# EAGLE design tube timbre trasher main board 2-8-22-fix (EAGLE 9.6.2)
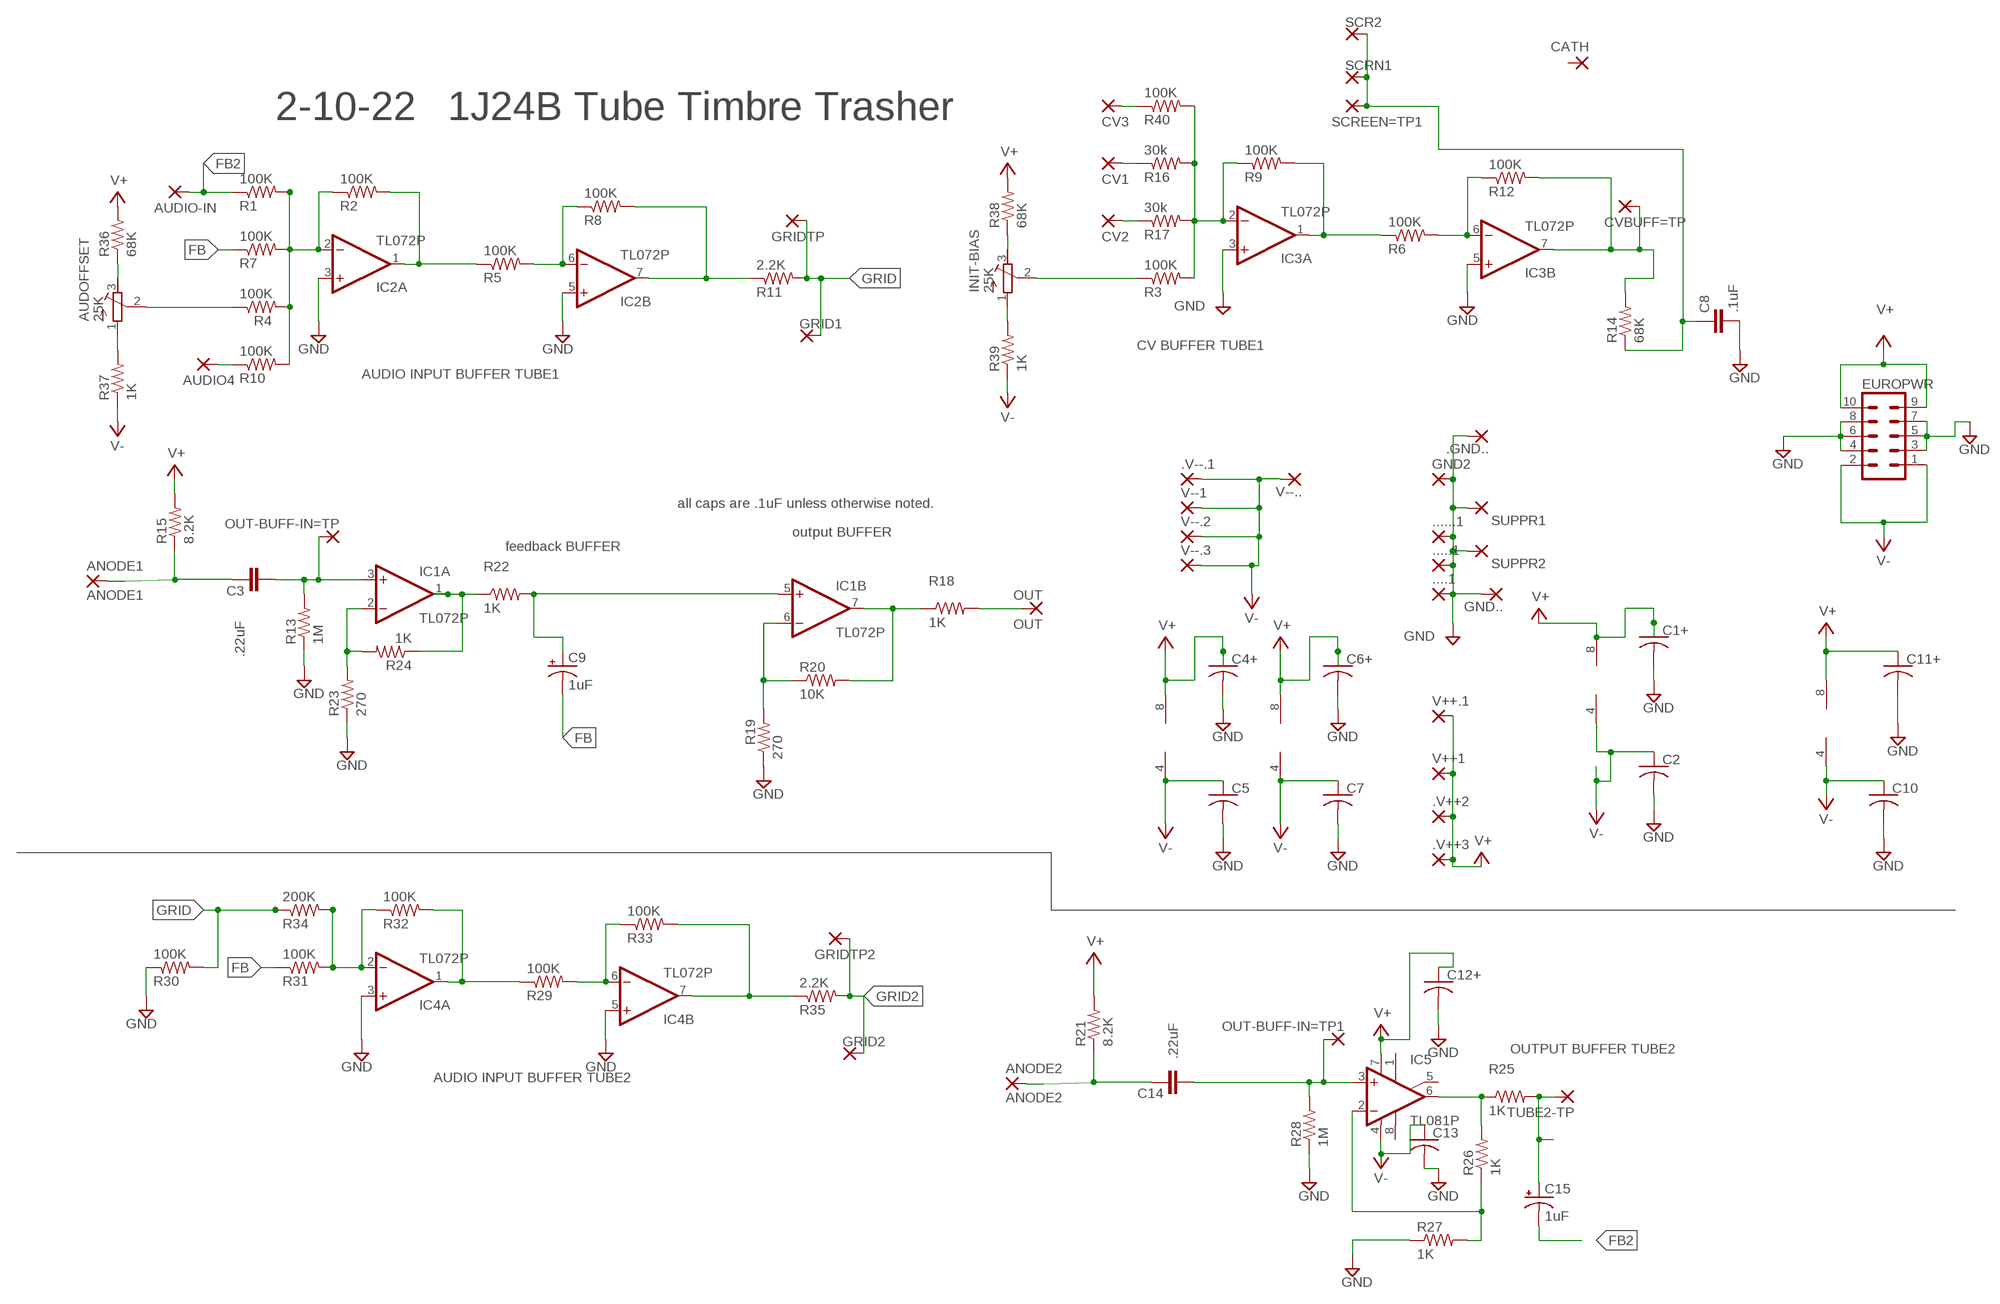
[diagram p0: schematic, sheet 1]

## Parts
....1  3,17/1,3  [3,17/1,3]
.....1  3,17/1,3  [3,17/1,3]
......1  3,17/1,3  [3,17/1,3]
.GND..  1  WIREPAD1,6/0,9  [1,6/0,9]
.V++2  2,54/1,0  [2,54/1,0]
.V++3  2,54/1,0  [2,54/1,0]
.V--.1  3,17/1,3  [3,17/1,3]
ANODE1  ANODE1  WIREPAD2,54/0,9  [2,54/0,9]
ANODE2  ANODE2  WIREPAD2,54/0,9  [2,54/0,9]
AUDIO4  3,17/1,3  [3,17/1,3]
AUDIO-IN  3,17/1,3  [3,17/1,3]
AUDOFFSET  25K  R-TRIMM64W  [RTRIM64W]
C1+  C-US025-025X050  [C025-025X050]
C2  C-US025-025X050  [C025-025X050]
C3  .22uF  C5/3.5  [C5B3.5]
C4+  C-US025-030X050  [C025-030X050]
C5  C-US025-025X050  [C025-025X050]
C6+  C-US025-025X050  [C025-025X050]
C7  C-US025-025X050  [C025-025X050]
C8  .1uF  C5/2.5  [C5B2.5]
C9  1uF  CPOL-USE2.5-6  [E2,5-6]
C10  C-US025-025X050  [C025-025X050]
C11+  C-US025-025X050  [C025-025X050]
C12+  C-US025-025X050  [C025-025X050]
C13  C-US025-025X050  [C025-025X050]
C14  .22uF  C5/3.5  [C5B3.5]
C15  1uF  CPOL-USE2.5-6  [E2,5-6]
CATH  1  WIREPAD1,6/0,9  [1,6/0,9]
CV1  3,17/1,3  [3,17/1,3]
CV2  3,17/1,3  [3,17/1,3]
CV3  3,17/1,3  [3,17/1,3]
CVBUFF=TP  3,17/1,3  [3,17/1,3]
EUROPWR  EURO_POWER_HEADERREGULAR  [EURO_POWER_HEADER]
GND2  3,17/1,3  [3,17/1,3]
GND..  1  WIREPAD1,6/0,9  [1,6/0,9]
GRID1  1  WIREPAD1,6/0,9  [1,6/0,9]
GRID2  1  WIREPAD1,6/0,9  [1,6/0,9]
GRIDTP  3,17/1,3  [3,17/1,3]
GRIDTP2  3,17/1,3  [3,17/1,3]
IC1  TL072P  [DIL08]
IC2  TL072P  [DIL08]
IC3  TL072P  [DIL08]
IC4  TL072P  [DIL08]
IC5  TL081P  [DIL08]
INIT-BIAS  25K  R-TRIMM64W  [RTRIM64W]
OUT  OUT  3,17/1,3  [3,17/1,3]
OUT-BUFF-IN=TP  3,17/1,3  [3,17/1,3]
OUT-BUFF-IN=TP1  3,17/1,3  [3,17/1,3]
R1  100K  R-US_0204/7  [0204/7]
R2  100K  R-US_0204/7  [0204/7]
R3  100K  R-US_0204/7  [0204/7]
R4  100K  R-US_0204/7  [0204/7]
R5  100K  R-US_0204/7  [0204/7]
R6  100K  R-US_0204/7  [0204/7]
R7  100K  R-US_0204/7  [0204/7]
R8  100K  R-US_0204/7  [0204/7]
R9  100K  R-US_0204/7  [0204/7]
R10  100K  R-US_0204/7  [0204/7]
R11  2.2K  R-US_0204/7  [0204/7]
R12  100K  R-US_0204/7  [0204/7]
R13  1M  R-US_0204/7  [0204/7]
R14  68K  R-US_0204/7  [0204/7]
R15  8.2K  R-US_0204/7  [0204/7]
R16  30k  R-US_0204/7  [0204/7]
R17  30k  R-US_0204/7  [0204/7]
R18  1K  R-US_0204/7  [0204/7]
R19  270  R-US_0204/7  [0204/7]
R20  10K  R-US_0204/7  [0204/7]
R21  8.2K  R-US_0207/7  [0207/7]
R22  1K  R-US_0204/7  [0204/7]
R23  270  R-US_0204/7  [0204/7]
R24  1K  R-US_0204/7  [0204/7]
R25  1K  R-US_0204/7  [0204/7]
R26  1K  R-US_0204/7  [0204/7]
R27  1K  R-US_0204/7  [0204/7]
R28  1M  R-US_0204/7  [0204/7]
R29  100K  R-US_0204/7  [0204/7]
R30  100K  R-US_0204/7  [0204/7]
R31  100K  R-US_0204/7  [0204/7]
R32  100K  R-US_0204/7  [0204/7]
R33  100K  R-US_0204/7  [0204/7]
R34  200K  R-US_0204/7  [0204/7]
R35  2.2K  R-US_0204/7  [0204/7]
R36  68K  R-US_0204/7  [0204/7]
R37  1K  R-US_0204/7  [0204/7]
R38  68K  R-US_0204/7  [0204/7]
R39  1K  R-US_0204/7  [0204/7]
R40  100K  R-US_0204/7  [0204/7]
SCR2  1  WIREPAD1,6/0,9  [1,6/0,9]
SCREEN=TP1  3,17/1,3  [3,17/1,3]
SCRN1  1  WIREPAD1,6/0,9  [1,6/0,9]
SUPPR1  1  WIREPAD1,6/0,9  [1,6/0,9]
SUPPR2  1  WIREPAD1,6/0,9  [1,6/0,9]
TUBE2-TP  3,17/1,3  [3,17/1,3]
V++1  2,54/1,0  [2,54/1,0]
V++.1  2,54/1,0  [2,54/1,0]
V--1  3,17/1,3  [3,17/1,3]
V--.2  3,17/1,3  [3,17/1,3]
V--.3  3,17/1,3  [3,17/1,3]
V--..  1  WIREPAD1,6/0,9  [1,6/0,9]

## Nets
FB: C9.- R7.1 R31.1
FB2: AUDIO-IN.1(P) C15.- R1.1
GND: ....1.1(P) .....1.1(P) ......1.1(P) .GND...1(P) C1+.2 C2.2 C4+.2 C5.2 C6+.2 C7.2 C8.2 C10.2 C11+.2 C12+.2 C13.2 EUROPWR.3 EUROPWR.4 EUROPWR.5 EUROPWR.6 EUROPWR.7 EUROPWR.8 GND2.1(P) GND...1(P) IC2.3(A:+IN) IC2.5(B:+IN) IC3.3(A:+IN) IC3.5(B:+IN) IC4.3(A:+IN) IC4.5(B:+IN) R13.1 R19.1 R23.1 R27.1 R28.1 R30.1 SUPPR1.1(P) SUPPR2.1(P)
GRID: GRID1.1(P) GRIDTP.1(P) R11.2 R30.2 R34.1
GRID2: GRID2.1(P) GRIDTP2.1(P) R35.2
N$1: ANODE1.1(P) C3.1 R15.1
N$2: C3.2 IC1.3(A:+IN) OUT-BUFF-IN=TP.1(P) R13.2
N$3: AUDOFFSET.3(E) R36.1
N$4: IC1.1(A:OUT) R22.1 R24.1
N$5: AUDOFFSET.1(A) R37.2
N$6: IC1.2(A:-IN) R23.2 R24.2
N$7: IC4.6(B:-IN) R29.2 R33.1
N$8: IC4.7(B:OUT) R33.2 R35.1
N$9: INIT-BIAS.3(E) R38.1
N$10: AUDOFFSET.2(S) R4.1
N$11: IC2.6(B:-IN) R5.2 R8.1
N$12: IC3.6(B:-IN) R6.2 R12.1
N$13: IC2.7(B:OUT) R8.2 R11.1
N$14: INIT-BIAS.1(A) R39.2
N$15: IC2.2(A:-IN) R1.2 R2.1 R4.2 R7.2 R10.2
N$16: IC2.1(A:OUT) R2.2 R5.1
N$17: CVBUFF=TP.1(P) IC3.7(B:OUT) R12.2 R14.2
N$19: IC4.2(A:-IN) R31.2 R32.1 R34.2
N$20: CV2.1(P) R17.1
N$21: IC3.2(A:-IN) R3.2 R9.1 R16.2 R17.2 R40.2
N$22: C15.+ R25.2 TUBE2-TP.1(P)
N$23: CV1.1(P) R16.1
N$24: IC4.1(A:OUT) R29.1 R32.2
N$25: INIT-BIAS.2(S) R3.1
N$26: IC1.6(B:-IN) R19.2 R20.1
N$27: C9.+ IC1.5(B:+IN) R22.2
N$28: AUDIO4.1(P) R10.1
N$29: IC1.7(B:OUT) R18.1 R20.2
N$30: OUT.1(P) R18.2
N$31: IC5.2(-IN) R26.1 R27.2
N$32: C14.2 IC5.3(+IN) OUT-BUFF-IN=TP1.1(P) R28.2
N$33: IC5.6(OUT) R25.1 R26.2
N$34: ANODE2.1(P) C14.1 R21.1
N$35: CV3.1(P) R40.1
TIE: C8.1 R14.1 SCR2.1(P) SCREEN=TP1.1(P) SCRN1.1(P)
TUBEBUS: IC3.1(A:OUT) R6.1 R9.2
V+: .V++2.1(P) .V++3.1(P) C1+.1 C4+.1 C6+.1 C11+.1 C12+.1 EUROPWR.9 EUROPWR.10 IC1.8(P:V+) IC2.8(P:V+) IC3.8(P:V+) IC4.8(P:V+) IC5.7(V+) R15.2 R21.2 R36.2 R38.2 V++1.1(P) V++.1.1(P)
V-: .V--.1.1(P) C2.1 C5.1 C7.1 C10.1 C13.1 EUROPWR.1 EUROPWR.2 IC1.4(P:V-) IC2.4(P:V-) IC3.4(P:V-) IC4.4(P:V-) IC5.4(V-) R37.1 R39.1 V--1.1(P) V--.2.1(P) V--.3.1(P) V--...1(P)
Unconnected: CATH.1(P) IC5.1(ON1) IC5.5(ON2) IC5.8(OPT)

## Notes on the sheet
- 2-10-22 | 1J24B Tube Timbre Trasher
- CV BUFFER TUBE1
- AUDIO INPUT BUFFER TUBE1
- all caps are .1uF unless otherwise noted.
- output BUFFER
- feedback BUFFER
- OUTPUT BUFFER TUBE2
- AUDIO INPUT BUFFER TUBE2

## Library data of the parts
....1 .....1 ......1 GND2 = wirepad:3,17/1,3: THROUGH-HOLE PAD
.GND.. CATH GND.. GRID1 GRID2 SCR2 SCRN1 SUPPR1 SUPPR2 V--.. = wirepad:WIREPAD: Wire PAD connect wire on PCB; SPICEPREFIX: X
.V++2 .V++3 V++1 V++.1 = wirepad-NONAMES:2,54/1,0: THROUGH-HOLE PAD
.V--.1 V--1 V--.2 V--.3 = wirepad-NONAMES:3,17/1,3: THROUGH-HOLE PAD
ANODE1 ANODE2 = wirepad:WIREPAD: Wire PAD connect wire on PCB
AUDIO4 AUDIO-IN CV1-CV3 CVBUFF=TP GRIDTP GRIDTP2 OUT OUT-BUFF-IN=TP OUT-BUFF-IN=TP1 SCREEN=TP1 TUBE2-TP = wirepad:3,17/1,3: THROUGH-HOLE PAD; SPICEPREFIX: X
AUDOFFSET INIT-BIAS = rcl:R-TRIMM: Trimm resistor; SPICEMODEL: X; SPICEPREFIX: J; SPICEPREFIXL: POT
C1+ C2 C4+ C5 C6+ C7 C10 C11+ C12+ C13 = rcl:C-US: CAPACITOR, American symbol; SPICEPREFIX: C
C3 C8 C14 = capacitor-wima:C: CAPACITOR; SPICEPREFIX: C
C9 C15 = rcl:CPOL-US: POLARIZED CAPACITOR, American symbol; SPICEPREFIX: C
EUROPWR = MusicThingModular:EURO_POWER_HEADER: Power Header 10 pin power header for Eurorack Power Supplies Variants with fatter pads for easier soldering, and the LOCK variant which has 5mil offset pins to hold the component in place before soldering
IC1 = linear:TL072: OP AMP
IC2-IC4 = linear:TL072: OP AMP; SPICEPREFIX: B
IC5 = linear:TL081: OP AMP; SPICEPREFIX: X
R1-R40 = rcl:R-US_: RESISTOR, American symbol; SPICEPREFIX: R

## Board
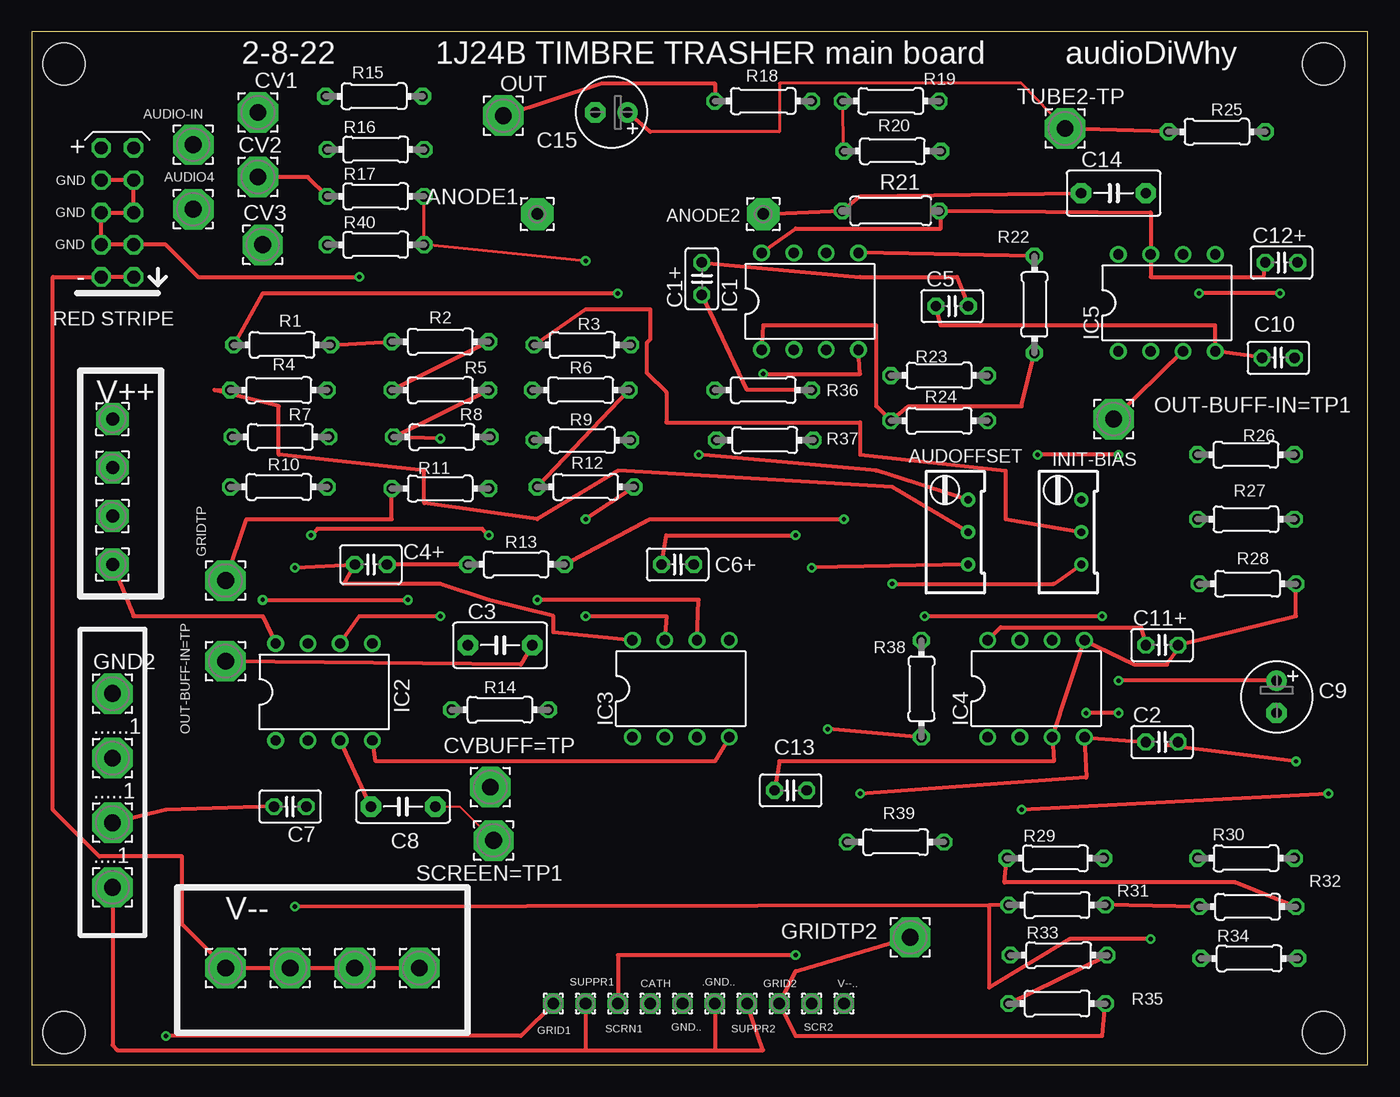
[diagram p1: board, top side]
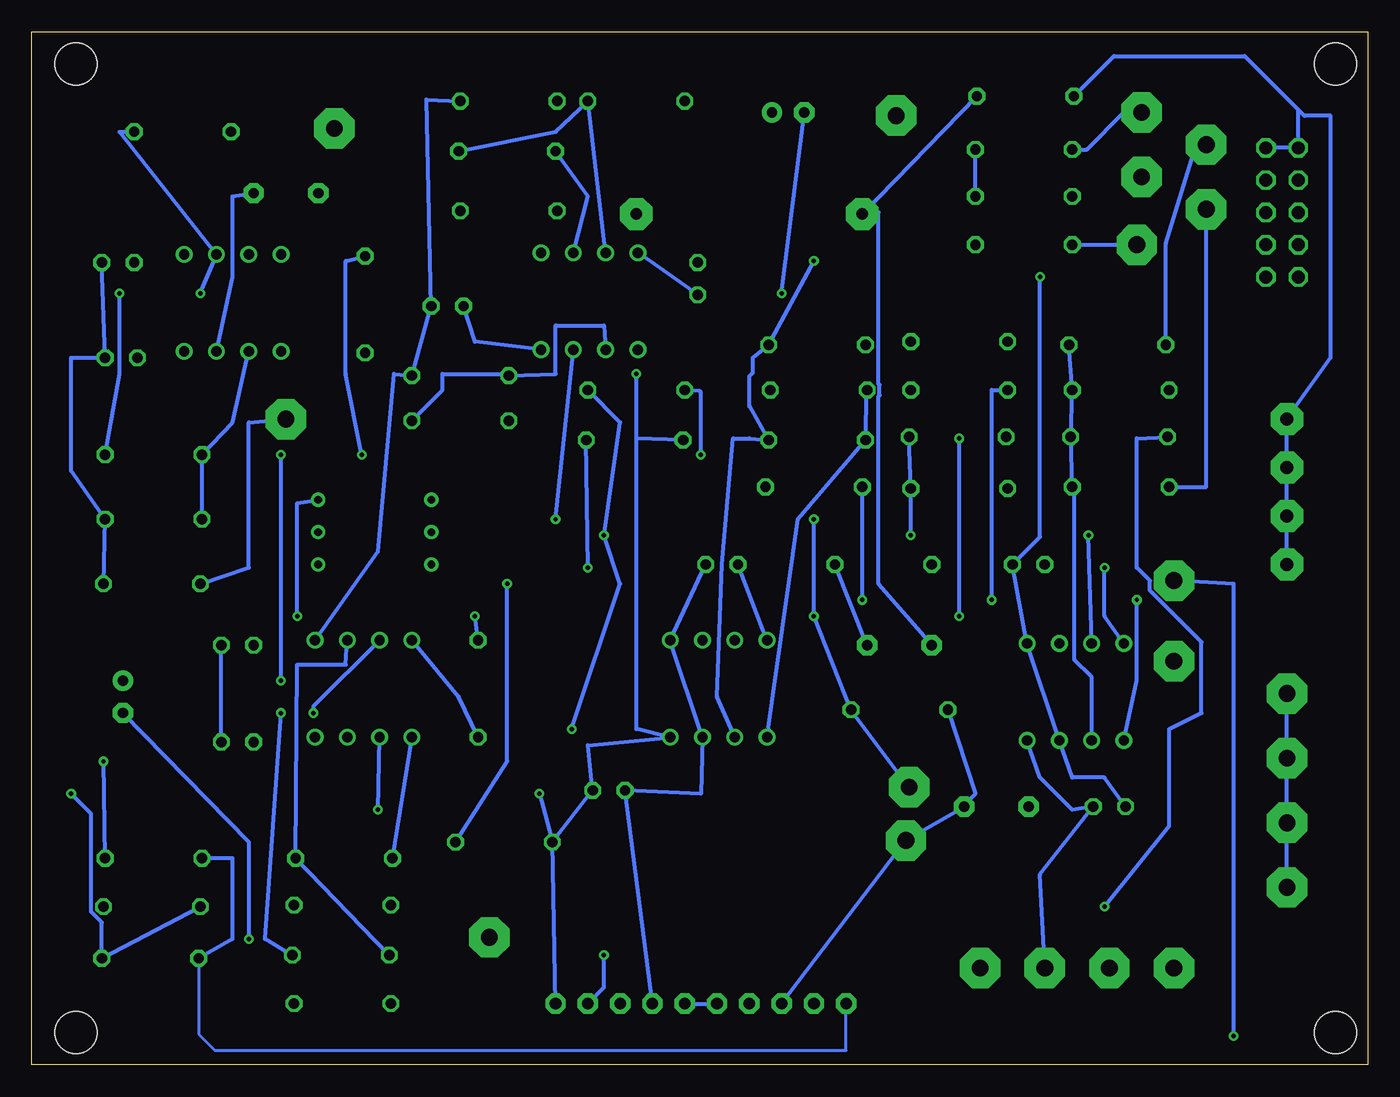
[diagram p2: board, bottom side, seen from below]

Size 105.08 x 81.27 mm. Coordinates in mm from the lower left corner, seen from the top.
Outline: 0,0 105.08,0 105.08,81.27 0,81.27 0,0
Copper layers (1*16): Top 0.035mm / dielectric 1.5mm / Bottom 0.035mm
Design rules "default": minimum track width 6mil, minimum drill 0.35mm, track to track 6mil, track to pad 6mil, pad to pad 6mil, via to via 6mil, smd to smd 6mil, copper to edge 40mil, drill to drill 6mil, minimum pad ring 10mil, minimum via ring 8mil, stop-mask expansion 4mil, vias tented up to drill 0mil, thermal gap 10mil
Holes 3.3 mm at 2.54,78.74 101.6,78.74 101.6,2.54 2.54,2.54

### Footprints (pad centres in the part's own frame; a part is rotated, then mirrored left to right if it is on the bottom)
3,17/1,3 = drill 1.321 pad 3.175 octagon: 1 0,0
1,6/0,9 = drill 0.914 pad 1.6 octagon: 1 0,0
2,54/1,0 = drill 1.016 pad 2.54 octagon: 1 0,0
2,54/0,9 = drill 0.914 pad 2.54 octagon: 1 0,0
RTRIM64W = drill 0.61: 1 1.27,-2.54; 2 1.27,0; 3 1.27,2.54
C025-025X050 = drill 0.813 octagon: 1 -1.27,0; 2 1.27,0
C5B3.5 = drill 0.813 pad 1.6 octagon: 1 -2.54,0; 2 2.54,0
C025-030X050 = drill 0.813 octagon: 1 -1.27,0; 2 1.27,0
C5B2.5 = drill 0.813 pad 1.6 octagon: 1 -2.54,0; 2 2.54,0
E2,5-6 = drill 0.813 pad 1.6: + -1.27,0 | drill 0.813 pad 1.6 octagon: - 1.27,0
EURO_POWER_HEADER = drill 1.016 octagon: 1 -5.08,-1.27; 2 -5.08,1.27; 3 -2.54,-1.27; 4 -2.54,1.27; 5 0,-1.27; 6 0,1.27; 7 2.54,-1.27; 8 2.54,1.27; 9 5.08,-1.27; 10 5.08,1.27
DIL08 = drill 0.813 pad 1.27: 1 -3.81,-3.81; 2 -1.27,-3.81; 3 1.27,-3.81; 4 3.81,-3.81; 5 3.81,3.81; 6 1.27,3.81; 7 -1.27,3.81; 8 -3.81,3.81
0204/7 = drill 0.813 octagon: 1 -3.81,0; 2 3.81,0
0207/7 = drill 0.813 octagon: 1 -3.81,0; 2 3.81,0

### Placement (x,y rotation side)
....1  6.35,13.97 0 top
.....1  6.35,19.05 0 top
......1  6.35,24.13 0 top
.GND..  53.72,4.83 0 top
.V++2  6.35,46.99 0 top
.V++3  6.35,39.37 0 top
.V--.1  15.24,7.62 0 top
ANODE1  39.75,66.93 0 top
ANODE2  57.53,66.93 0 top
AUDIO4  12.7,67.31 0 top
AUDIO-IN  12.7,72.39 0 top
AUDOFFSET  72.39,41.91 0 top
C1+  52.7,61.85 90 top
C2  88.9,25.4 0 top
C3  36.83,33.02 0 top
C4+  26.67,39.37 0 top
C5  72.39,59.69 0 top
C6+  50.8,39.37 0 top
C7  20.32,20.32 180 top
C8  29.21,20.32 180 top
C9  97.92,28.96 270 top
C10  98.04,55.63 0 top
C11+  88.9,33.02 0 top
C12+  98.3,63.12 0 top
C13  59.69,21.59 180 top
C14  85.09,68.58 0 top
C15  45.59,74.93 180 top
CATH  48.64,4.83 0 top
CV1  17.78,74.93 0 top
CV2  17.78,69.85 0 top
CV3  18.16,64.52 0 top
CVBUFF=TP  36.07,21.84 0 top
EUROPWR  6.73,67.06 90 top
GND2  6.35,29.21 0 top
GND..  51.18,4.83 0 top
GRID1  41.02,4.83 0 top
GRID2  58.8,4.83 0 top
GRIDTP  15.24,38.1 0 top
GRIDTP2  69.09,10.03 0 top
IC1  61.21,60.07 0 top
IC2  22.99,29.34 0 top
IC3  51.05,29.59 0 top
IC4  78.99,29.59 0 top
IC5  89.28,59.94 0 top
INIT-BIAS  81.28,41.91 0 top
OUT  37.08,74.68 0 top
OUT-BUFF-IN=TP  15.24,31.75 0 top
OUT-BUFF-IN=TP1  85.09,50.8 0 top
R1  19.68,56.64 0 top
R2  32.13,56.9 0 top
R3  43.31,56.64 0 top
R4  19.43,53.09 0 top
R5  32.13,53.09 0 top
R6  43.18,53.09 0 top
R7  19.56,49.4 0 top
R8  32.26,49.4 0 top
R9  43.31,49.15 180 top
R10  19.43,45.47 0 top
R11  32.13,45.34 180 top
R12  43.56,45.47 0 top
R13  38.1,39.37 0 top
R14  36.83,27.94 0 top
R15  26.92,76.2 180 top
R16  27.05,72.01 0 top
R17  27.05,68.33 0 top
R18  57.53,75.82 180 top
R19  67.56,75.82 180 top
R20  67.69,71.88 0 top
R21  67.56,67.18 0 top
R22  78.87,59.82 90 top
R23  71.37,54.23 180 top
R24  71.37,50.67 0 top
R25  93.22,73.41 180 top
R26  95.5,48.01 0 top
R27  95.5,42.93 180 top
R28  95.63,37.85 180 top
R29  80.52,16.26 0 top
R30  95.5,16.26 180 top
R31  80.64,12.57 0 top
R32  95.63,12.45 0 top
R33  80.77,8.64 0 top
R34  95.76,8.38 0 top
R35  80.64,4.83 0 top
R36  57.53,53.09 0 top
R37  57.66,49.15 0 top
R38  69.98,29.59 270 top
R39  67.94,17.53 0 top
R40  27.05,64.52 0 top
SCR2  61.34,4.83 0 top
SCREEN=TP1  36.32,17.65 0 top
SCRN1  46.1,4.83 0 top
SUPPR1  43.56,4.83 0 top
SUPPR2  56.26,4.83 0 top
TUBE2-TP  81.28,73.66 0 top
V++1  6.35,50.8 0 top
V++.1  6.35,43.18 0 top
V--1  30.48,7.62 0 top
V--.2  20.32,7.62 0 top
V--.3  25.4,7.62 0 top
V--..  63.88,4.83 0 top

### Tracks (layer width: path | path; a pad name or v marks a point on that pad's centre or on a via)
FB  (via drill 0.35)
  Top 0.305: R31.1 75.31,12.57 | 75.31,12.57 v20.7,12.45 | v88.01,9.91 81.66,9.91 75.31,6.1 75.31,12.57
  Bottom 0.305: v20.7,12.45 15.62,18.8 15.62,26.42 13.08,27.69 13.08,33.27 17.13,37.32 17.13,38.09 18.16,39.12 18.16,49.28 R7.1 | C9.- 88.01,17.53 v88.01,9.91
FB2  (via drill 0.35)
  Top 0.305: R1.1 18.16,60.71 v46.1,60.71
  Bottom 0.305: R1.1 15.88,64.61 13.85,71.24 AUDIO-IN.1 | v46.1,60.71 C15.-
GND  (via drill 0.35)
  Top 0.305: C7.2 10.54,20.07 .....1.1 | R13.1 C4+.2 | ....1.1 6.35,1.55 6.73,1.17 43.56,1.17 | 43.56,1.17 53.72,1.17 | 53.72,1.17 57.53,1.17 SUPPR2.1 | C8.2 IC2.3 | C11+.2 90.47,33.09 | 90.47,33.09 99.44,35.31 R28.1 | v99.44,23.88 89.28,25.15 C2.2 | C13.2 58.8,23.88 80.39,23.88 IC4.3 IC4.5 86.74,31.5 89.28,31.5 90.47,33.09 | C1+.2 65.15,61.98 72.77,61.98 C5.2 | SUPPR1.1 43.56,1.17 | .GND...1 53.72,1.17 | EUROPWR.8 EUROPWR.7 EUROPWR.5 EUROPWR.6 EUROPWR.4 EUROPWR.3 10.54,64.52 13.08,61.98 v25.78,61.98
  Bottom 0.305: ....1.1 .....1.1 ......1.1 GND2.1 | .GND...1 GND...1 | C7.2 20.7,22.61 23.24,22.61 IC2.3 IC2.5 C4+.2 25.78,41.53 v25.78,61.98 | SUPPR2.1 C13.2 52.45,21.34 IC3.3 IC3.5 C6+.2 | R19.1 74.04,75.95 C5.2 R23.1 76.58,54.36 77.85,40.39 IC4.5 | C2.2 C11+.2 | R28.1 R27.1 101.98,46.74 101.98,55.63 C10.2 C12+.2 | R30.1 v99.44,23.88
GRID  (via drill 0.35)
  Top 0.305: GRID1.1 38.48,2.29 v10.54,2.29 | GRIDTP.1 16.89,42.93 28.32,42.93 R11.2
  Bottom 0.254: R34.1 91.95,2.41 90.68,1.14 41.02,1.14 GRID1.1
  Bottom 0.305: v10.54,2.29 10.54,37.85 GRIDTP.1 | R34.1 89.28,9.91 89.28,16.26 R30.2
GRID2
  Top 0.305: GRIDTP2.1 60.07,7.37 GRID2.1 60.07,2.29 84.2,2.29 R35.2
N$1
  Bottom 0.305: R15.1 ANODE1.1 38.48,67.06 38.48,53.56 38.41,53.49 38.41,52.69 38.48,52.61 38.48,37.85 C3.1
N$2  (via drill 0.35)
  Top 0.305: C3.2 38.48,31.5 OUT-BUFF-IN=TP.1 | R13.2 48.64,42.93 v63.88,42.93
  Bottom 0.305: C3.2 R13.2 | v63.88,42.93 IC1.3
N$3  (via drill 0.35)
  Top 0.305: AUDOFFSET.3 66.42,46.74 v52.45,48.01
  Bottom 0.305: v52.45,48.01 52.45,52.91 52.54,53 R36.1
N$4
  Top 0.305: R22.1 77.85,51.82 68.96,51.82 R24.1 66.42,51.82 66.42,58.17 57.53,58.17 IC1.1
N$5  (via drill 0.35)
  Top 0.305: AUDOFFSET.1 v61.34,39.12
  Bottom 0.305: v61.34,39.12 R37.2
N$6
  Bottom 0.305: IC1.2 60.07,58.17 63.88,58.17 63.88,54.36 R23.2 67.69,54.36 72.77,54.36 72.77,53.09 R24.2
N$7
  Bottom 0.305: R33.1 R29.2 84.2,31.5 80.39,31.5 IC4.6
N$8  (via drill 0.35)
  Top 0.305: R35.1 R33.2 | v85.47,27.69 v82.93,27.69
  Bottom 0.305: R33.2 86.74,9.91 v85.47,27.69 | IC4.7 82.93,28.19 v82.93,27.69
N$9  (via drill 0.35)
  Top 0.305: v70.23,35.31 v84.2,35.31
  Bottom 0.305: R38.1 v70.23,35.31 | v84.2,35.31 84.2,44.2 INIT-BIAS.3
N$10
  Top 0.305: AUDOFFSET.2 67.69,45.47 46.1,46.74 39.75,42.93 30.86,44.2 30.86,46.74 19.43,48.01 19.43,51.82 14.35,53.09 R4.1
N$11  (via drill 0.35)
  Top 0.305: R5.2 R8.1 v32.13,49.28 | IC2.6 25.78,35.31 v32.13,35.31
  Bottom 0.305: v32.13,35.31 v32.13,49.28
N$12  (via drill 0.35)
  Top 0.305: IC3.6 52.45,36.58 v39.75,36.58 | R12.1 R6.2
  Bottom 0.305: v39.75,36.58 R12.1
N$13  (via drill 0.35)
  Top 0.305: v21.97,41.66 22.48,42.16 35.43,42.16 v35.94,41.66
  Bottom 0.305: IC2.7 v21.97,41.66 | v35.94,41.66 R11.1 R8.2
N$14  (via drill 0.35)
  Top 0.305: v67.69,37.85 80.39,37.85 INIT-BIAS.1
  Bottom 0.305: R39.2 67.69,23.88 v67.69,37.85
N$15
  Top 0.305: R1.2 R2.1
  Bottom 0.305: R1.2 R4.2 R7.2 R10.2 23.06,45.29 23.06,31.86 21.72,30.51 IC2.2
N$16  (via drill 0.35)
  Top 0.305: R5.1 R2.2 | v18.16,36.58 v29.59,36.58
  Bottom 0.305: IC2.1 18.16,30.23 v18.16,36.58 | v29.59,36.58 29.59,53.09 R5.1
N$17  (via drill 0.35)
  Top 0.305: v43.56,35.31 49.91,35.31 IC3.7 | v43.56,42.93 R12.2
  Bottom 0.305: CVBUFF=TP.1 R14.2 v43.56,35.31 v43.56,42.93
N$19  (via drill 0.35)
  Top 0.305: R32.1 R31.2 | v101.98,21.34 v77.85,20.07
  Bottom 0.305: R32.1 R34.2 99.57,11.21 100.41,12.05 100.41,19.76 v101.98,21.34 | v77.85,20.07 IC4.2
N$20
  Top 0.305: R17.1 21.72,69.85 CV2.1
N$21  (via drill 0.35)
  Top 0.254: v43.56,63.25 R40.2 R17.2
  Bottom 0.305: R17.2 R16.2 | v43.56,63.25 R3.2 48.36,55.63 48.36,54.46 48.64,54.18 48.64,51.82 R9.1 48.64,49.28 49.91,49.28 50.8,39.37 51.18,28.96 IC3.2
N$22
  Top 0.254: TUBE2-TP.1 77.85,77.22 58.8,77.22 58.8,73.41 48.64,73.41
  Top 0.305: R25.2 TUBE2-TP.1 | 48.64,73.41 C15.+
N$23
  Bottom 0.305: R16.1 22.1,72.01 19.18,74.93 CV1.1
N$24
  Top 0.305: R32.2 94.68,14.35 76.52,14.35 R29.1
  Bottom 0.305: R29.1 IC4.1
N$25
  Top 0.305: R3.1 43.56,59.44 48.64,59.44 48.64,57.07 48.36,56.79 48.36,54.46 49.91,52.91 49.91,50.55 65.15,50.55 65.15,48.01 76.58,46.74 76.58,42.93 INIT-BIAS.2
N$26
  Top 0.254: R20.1 R19.2
  Bottom 0.305: IC1.6 61.34,68.33 R20.1
N$27  (via drill 0.35)
  Top 0.305: R22.2 IC1.5 | C9.+ v85.47,30.23 | v85.47,48.01 v79.12,48.01
  Bottom 0.305: v85.47,30.23 v85.47,48.01 | v79.12,48.01 80.39,54.36 80.39,63.25 R22.2
N$28
  Bottom 0.305: R10.1 12.7,45.47 AUDIO4.1
N$29
  Bottom 0.305: IC1.7 R18.1 63.88,73.41 R20.2
N$30
  Top 0.305: OUT.1 44.83,77.22 53.72,77.22 R18.2
N$31
  Bottom 0.305: IC5.2 89.28,50.55 R26.1 R27.2
N$32
  Top 0.305: OUT-BUFF-IN=TP1.1 IC5.3
  Bottom 0.305: IC5.3 89.28,61.98 89.28,68.33 C14.2 | R28.2 88.01,39.12 88.01,50.55 OUT-BUFF-IN=TP1.1
N$33  (via drill 0.35)
  Top 0.305: v98.17,60.71 v91.82,60.71
  Bottom 0.305: R25.1 98.17,73.41 IC5.6 v91.82,60.71 | R26.2 98.17,54.36 v98.17,60.71
N$34
  Top 0.305: ANODE2.1 R21.1 65.15,68.33 C14.1
N$35
  Bottom 0.305: R40.1 CV3.1
TIE  (via drill 0.35)
  Top 0.152: C8.1 33.66,20.32 SCREEN=TP1.1
  Top 0.305: v60.07,8.64 46.1,8.64 SCRN1.1
  Bottom 0.305: SCRN1.1 SCREEN=TP1.1 32.13,20.07 30.86,21.34 R14.1 | SCR2.1 60.07,6.1 v60.07,8.64
TUBEBUS
  Bottom 0.305: IC3.1 44.83,42.93 R9.2 R6.1
V+  (via drill 0.35)
  Top 0.305: .V++3.1 8,35.31 18.16,35.31 IC2.8 | v20.7,39.12 C4+.1 24.51,37.85 32.13,37.85 35.94,36.58 41.02,35.31 41.02,34.04 IC3.8 | R21.2 71.5,67.18 | 71.5,67.18 88.01,67.06 IC5.7 88.01,61.98 96.9,61.98 C12+.1 | C6+.1 49.91,41.66 v60.07,41.66 | R38.2 v62.61,26.42 | IC1.8 60.07,65.79 71.5,65.79 71.5,67.18 | R36.2 56.26,53.09 C1+.1 | IC4.8 76.2,34.42 87.25,34.42 C11+.1
  Bottom 0.305: 5.46,75.13 4.98,74.65 2.92,74.65 2.92,55.63 V++1.1 .V++2.1 V++.1.1 .V++3.1 | R15.2 19.96,79.35 9.68,79.35 5.46,75.13 | IC2.8 20.7,35.31 v20.7,39.12 | R38.2 71.5,28.96 IC4.8 | IC3.8 C6+.1 | R36.2 58.8,50.55 v60.07,41.66 58.8,37.85 v62.61,26.42 | C1+.1 IC1.8 | EUROPWR.9 EUROPWR.10 5.46,75.13
V-  (via drill 0.35)
  Top 0.305: IC3.4 53.72,23.88 27.05,23.88 IC2.4 | C2.1 IC4.4 82.93,22.61 v65.15,21.34 | C10.1 IC5.4 93.09,58.17 71.5,58.17 C5.1 | v57.53,54.36 65.15,54.36 IC1.4 | V--1.1 V--.3.1 V--.2.1 .V--.1.1 11.81,11.05 11.81,16.4 5.32,16.4 1.65,20.07 1.65,61.98 EUROPWR.2 EUROPWR.1
  Bottom 0.305: V--.3.1 25.78,14.99 C7.1 23.24,20.07 25.78,22.61 IC2.4 | V--...1 R39.1 | R39.1 C13.1 61.34,25.15 IC3.4 57.53,26.42 57.53,49.28 | R37.1 57.53,49.28 | v65.15,21.34 R39.1 | 57.53,49.28 v57.53,54.36 | IC1.4 70.23,56.9 C5.1

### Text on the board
tNames: 2-8-22 | 1J24B TIMBRE TRASHER main board | audioDiWhy | V++ | V--
tValues: V-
